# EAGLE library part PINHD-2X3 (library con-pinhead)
PIN HEADER
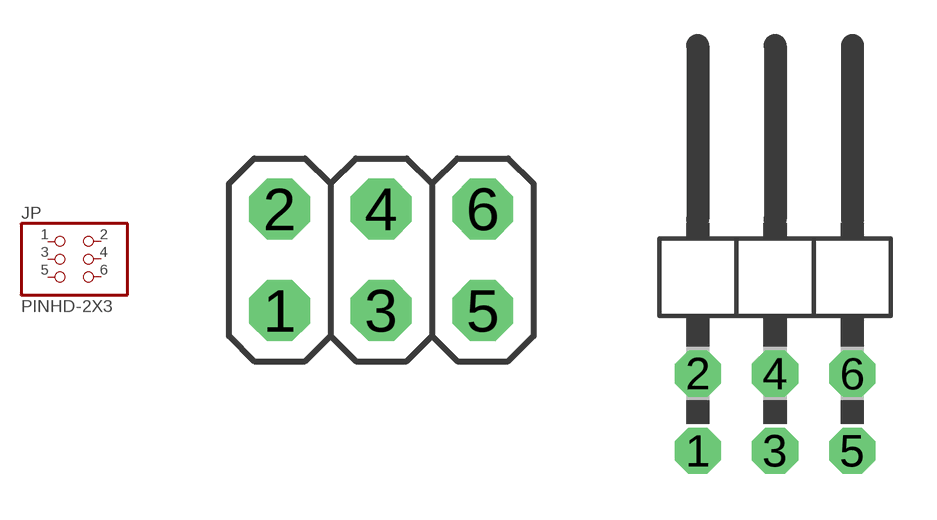
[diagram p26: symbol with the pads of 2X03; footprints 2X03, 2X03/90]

Designator prefix JP

## PINHD-2X3_2.54  [2X03]
1  1  pas
2  2  pas
3  3  pas
4  4  pas
5  5  pas
6  6  pas

## PINHD-2X3_2.54-90°  [2X03/90]
Pads as for 2X03

## PINHD-2X3_2.00  [2X03M]
Pads as for 2X03

## PINHD-2X3_2.54-SMD  [2X03SMD]
Pads as for 2X03

## PINHD-2X3_MICROMATCH  [MICROMATCH-6]
Pads as for 2X03

## PINHD-2X3_2.54-SMD-90°  [2X03SMD/90]
Pads as for 2X03

## Footprint 2X03 (pad centres in mm)
PIN HEADER - 2.54
drill 1.016 octagon: 1 -2.54,-1.27; 2 -2.54,1.27; 3 0,-1.27; 4 0,1.27; 5 2.54,-1.27; 6 2.54,1.27

## Footprint 2X03/90 (pad centres in mm)
PIN HEADER - 2.54 90°
drill 1.016 octagon: 1 -2.54,-6.35; 2 -2.54,-3.81; 3 0,-6.35; 4 0,-3.81; 5 2.54,-6.35; 6 2.54,-3.81

## Footprint 2X03M (pad centres in mm)
PIN HEADER - 2
drill 0.914 square: 1 -2,-1
drill 0.914: 2 -2,1; 3 0,-1; 4 0,1; 5 2,-1; 6 2,1

## Footprint 2X03SMD (pad centres in mm)
PIN HEADER - 2.54 SMD
smd 1.016 x 3.302: 1 -2.54,-2.54; 2 -2.54,2.54; 3 0,-2.54; 4 0,2.54; 5 2.54,-2.54; 6 2.54,2.54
